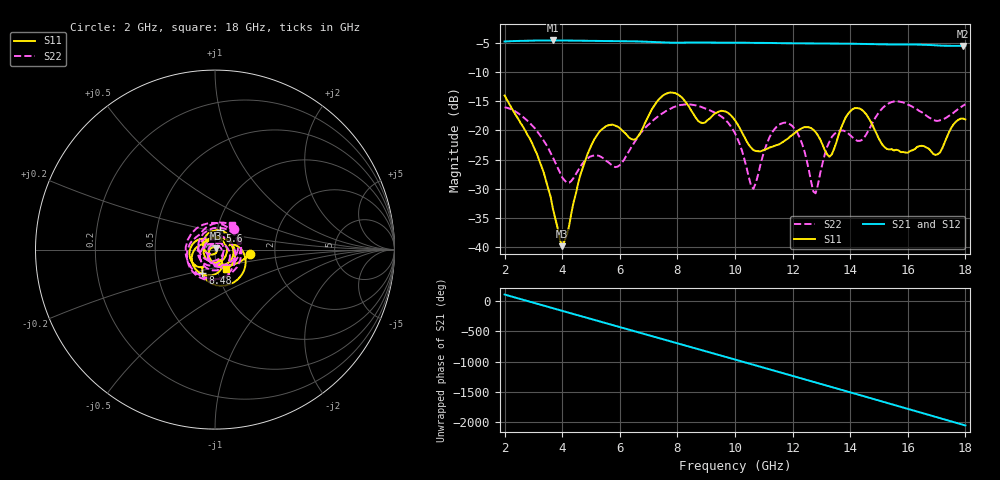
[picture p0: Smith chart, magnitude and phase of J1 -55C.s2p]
!Agilent Technologies,E8363B,SG43030131,A.07.50.48
!Agilent E8363B: A.07.50.48
!Date: Wednesday, December 17, 2025 22:27:25
!Correction: S11(Full 2 Port(1,2))
!S21(Full 2 Port(1,2))
!S12(Full 2 Port(1,2))
!S22(Full 2 Port(1,2))
!S2P File: Measurements: S11, S21, S12, S22:
# Hz S  dB  R 50
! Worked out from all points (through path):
!   201 points, 2 GHz to 18 GHz, reference 50 ohm
!   highest |S21| = -4.64 dB at 3.68 GHz (marker M1); lowest = -5.6 dB at 17.92 GHz (marker M2)
!   group delay of S21, straight-line fit = 372 ps
!   lowest |S11| = -39.8 dB at 4 GHz (marker M3), VSWR 1.02, Z = 50.7 + j0.777 ohm
!   |S11| at or under -10 dB: start of sweep to end of sweep
!   |S22| runs from -30.7 to -15.1 dB; largest |S21 - S12| = 0.0022
!   S11 on the Smith chart (normalised r, x): 2 GHz: 1.49, -0.07; 5.6 GHz: 1.03, +0.22; 8.48 GHz: 0.84, -0.22; 18 GHz: 1.10, -0.24
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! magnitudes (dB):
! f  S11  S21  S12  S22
! 2 GHz  -14.0  -4.8  -4.8  -16.1
! 3.12 GHz  -24.0  -4.6  -4.7  -20.1
! 3.68 GHz  -33.4  -4.6  -4.6  -24.6
! 4 GHz  -39.8  -4.6  -4.6  -28.0
! 4.72 GHz  -26.3  -4.7  -4.7  -25.6
! 5.6 GHz  -19.1  -4.7  -4.7  -25.4
! 6.56 GHz  -21.5  -4.8  -4.8  -21.6
! 7.36 GHz  -14.7  -5.0  -5.0  -17.5
! 8.48 GHz  -16.6  -5.0  -5.0  -15.6
! 10 GHz  -18.3  -5.0  -5.0  -20.5
! 10.64 GHz  -23.4  -5.0  -5.0  -30.0
! 11.28 GHz  -22.8  -5.1  -5.1  -20.4
! 11.92 GHz  -21.0  -5.1  -5.1  -19.0
! 12.32 GHz  -19.6  -5.1  -5.1  -22.2
! 12.72 GHz  -19.9  -5.2  -5.2  -30.4
! 13.28 GHz  -24.5  -5.2  -5.2  -21.9
! 13.84 GHz  -17.8  -5.2  -5.2  -20.2
! 14.32 GHz  -16.2  -5.2  -5.2  -21.8
! 15.36 GHz  -23.2  -5.3  -5.3  -15.3
! 17.04 GHz  -24.1  -5.5  -5.5  -18.4
! 17.92 GHz  -18.0  -5.6  -5.6  -15.8
! 18 GHz  -18.1  -5.6  -5.6  -15.5
